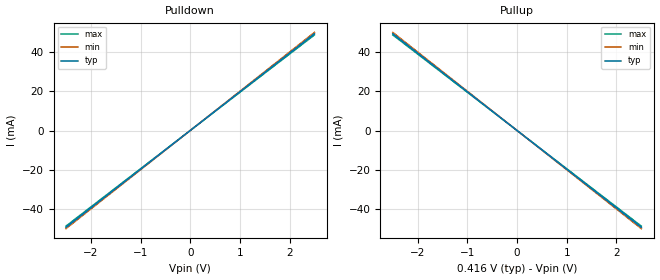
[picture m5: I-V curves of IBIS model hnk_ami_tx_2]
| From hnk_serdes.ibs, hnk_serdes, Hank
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|   model   hnk_ami_tx_2
[Model] hnk_ami_tx_2
Model_type Output
C_comp 800f 750f 850f
Cref = 0
[Model Spec]
Vmeas .208 .198 .218
Vref .208 .198 .218
[Temperature Range]  25 100 0
[Voltage Range] .416 .395 .436
[Algorithmic Model]
Executable Windows_VisualStudio7.1.3088_64 hnkffe.dll hnkffe.ami
Executable Linux_gcc3.2.3_64 hnkffe.linux.so hnkffe.ami
[End Algorithmic Model]
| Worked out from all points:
|   slope of the pulldown table from 0 to 0.062 V, typ, clamps not added: 50.4 ohm
|   slope of the pullup table from 0 to 0.062 V, typ, clamps not added: 50.4 ohm
[Pulldown]
-2.5V     -49.6mA    -50.26mA   -48.96mA
0V        0A         0A         0A
2.5V      49.6mA     50.26mA    48.96mA
[Pullup]
-2.5V     49.6mA     50.26mA    48.96mA
0V        0A         0A         0A
2.5V      -49.6mA    -50.26mA   -48.96mA
[Ramp]
dV/dt_r .124/60f .119/60f .129/60f
dV/dt_f .124/60f .119/60f .129/60f
